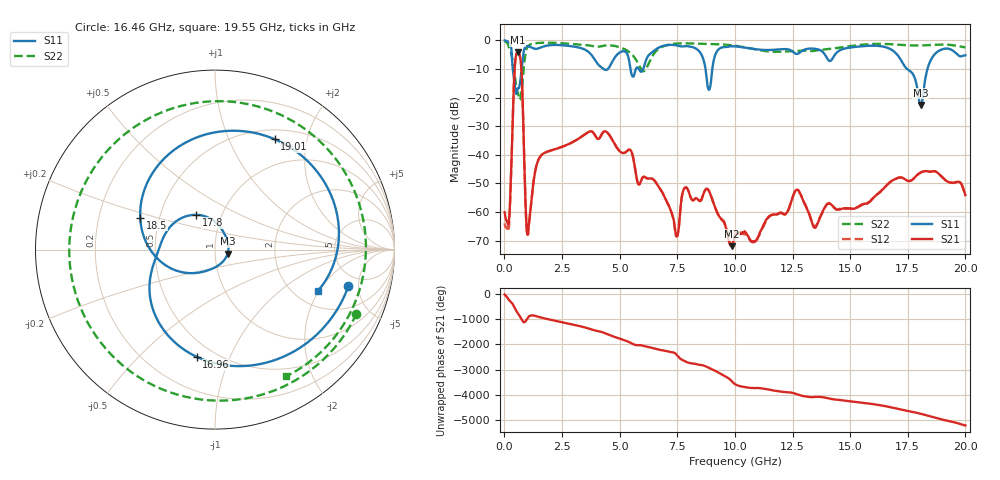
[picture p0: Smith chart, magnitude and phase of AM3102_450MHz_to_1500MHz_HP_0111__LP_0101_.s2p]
!Agilent Technologies,E8364B,MY43040894,A.07.50.67
!Agilent E8364B: A.07.50.67
!Date: Thursday, January 11, 2018 05:52:11
!Correction: S11(Full 2 Port(1,2))
!S21(Full 2 Port(1,2))
!S12(Full 2 Port(1,2))
!S22(Full 2 Port(1,2))
!S2P File: Measurements: S11, S21, S12, S22:
# Hz S  dB  R 50
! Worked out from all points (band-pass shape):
!   1601 points, 10 MHz to 20 GHz, reference 50 ohm
!   highest |S21| = -4.26 dB at 584.7 MHz (marker M1); lowest = -71.9 dB at 9.855 GHz (marker M2)
!   |S21| within 3 dB of the highest: 471.6 MHz to 708.7 MHz (237 MHz wide, 40.2 % of centre)
!   lowest |S11| = -22.6 dB at 18.06 GHz (marker M3), VSWR 1.16, Z = 57.5 - j2.59 ohm
!   |S11| at or under -10 dB: 365.5 MHz to 748.5 MHz (382.9 MHz wide, 68.7 % of centre); 8.724 GHz to 9.02 GHz (296.4 MHz wide, 3.34 % of centre); 17.47 GHz to 18.36 GHz (890.1 MHz wide, 4.97 % of centre)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
!   |S22| runs from -20.8 to -0.4 dB; largest |S21 - S12| = 0.0018
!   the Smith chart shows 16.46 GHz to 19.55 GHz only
!   S11 on the Smith chart (normalised r, x): 16.46 GHz: 3.80, -3.80; 16.96 GHz: 0.40, -0.76; 17.8 GHz: 0.76, +0.31; 18.5 GHz: 0.39, +0.17; 19.01 GHz: 0.62, +1.49; 19.55 GHz: 2.62, -1.95
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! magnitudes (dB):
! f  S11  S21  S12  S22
! 10 MHz  -0.1  -60.1  -63.9  -0.4
! 197.4 MHz  -0.7  -63.1  -65.2  -2.5
! 584.7 MHz  -16.8  -4.3  -4.3  -18.1
! 1.022 GHz  -2.0  -67.6  -68.0  -2.1
! 1.534 GHz  -2.7  -40.9  -40.9  -0.9
! 3.346 GHz  -2.8  -33.7  -33.6  -1.5
! 6.682 GHz  -2.6  -51.0  -51.0  -3.1
! 7.469 GHz  -1.8  -68.5  -68.5  -1.1
! 8.881 GHz  -17.3  -52.7  -52.6  -1.3
! 9.855 GHz  -2.1  -71.9  -71.4  -1.7
! 10.01 GHz  -2.1  -68.8  -67.7  -1.9
! 12.69 GHz  -4.8  -52.2  -52.1  -3.7
! 13.34 GHz  -2.9  -63.7  -63.2  -3.8
! 16.46 GHz  -2.3  -51.7  -51.6  -1.3
! 16.68 GHz  -2.8  -49.9  -49.9  -1.3
! 16.96 GHz  -4.3  -48.5  -48.5  -1.5
! 17.8 GHz  -13.1  -47.9  -47.9  -1.8
! 18.06 GHz  -22.6  -46.2  -46.2  -1.8
! 18.5 GHz  -6.9  -45.9  -45.9  -1.7
! 19.01 GHz  -3.1  -48.0  -48.0  -1.5
! 19.55 GHz  -4.2  -49.7  -49.6  -1.8
! 20 GHz  -5.2  -54.1  -54.4  -2.4
